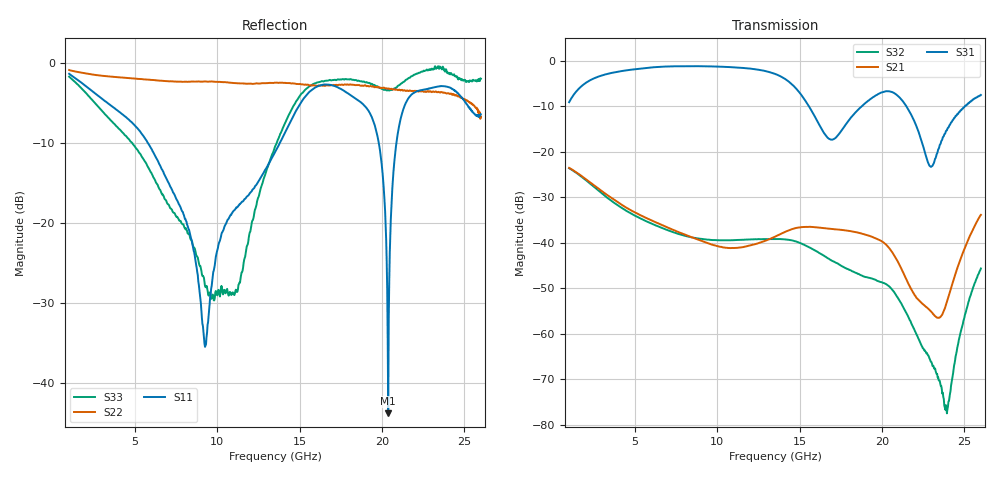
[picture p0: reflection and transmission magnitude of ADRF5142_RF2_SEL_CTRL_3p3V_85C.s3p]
! Device: ADRF5142
! Description: Silicon, SPDT Switch, Reflective
! Frequency: 8.00 GHz - 11.00 GHz
! Ports:
!  RFC = Port 1
!  RF1 = Port 2
!  RF2 = Port 3
! VDD = +3.3V
! VSS = -3.3V
! CTRL = +3.3V
! Temp = 85C
! Data:  Data was collected using an calibrated 4 port network analyzer.
!  The reference plane is the package pins of ADRF5142 switch.
! Notes: Analog Devices supplies this data as a sample of measured data
!  for this product.  Your particular data for this product may vary.
!  Data was taken at 85 degrees C.
!  Analog Devices reserves the right to change this data at anytime.
# HZ S DB R 50
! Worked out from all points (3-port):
!   801 points, 1 GHz to 26 GHz, reference 50 ohm
!   strongest paths, dB at 1 GHz, 7.25 GHz, 13.5 GHz, 19.75 GHz, 26 GHz:
!     S31: -9.1, -1.2, -2.9, -7.3, -7.5
!     S21: -23.5, -37.0, -38.6, -39.2, -33.9
!     S32: -23.6, -37.6, -39.2, -48.4, -45.6
!   lowest |S11| = -43.8 dB at 20.38 GHz (marker M1), VSWR 1.01, Z = 50.2 - j0.611 ohm
!   |S11| at or under -10 dB: 5.768 GHz to 13.8 GHz (8.035 GHz wide, 82.1 % of centre); 19.8 GHz to 20.87 GHz (1.075 GHz wide, 5.29 % of centre)
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1e9  -1.40 158.2  -23.53 -37.4  -9.09 36.3
     -23.53 -37.4  -0.93 171.1  -23.60 -55.0
     -9.09 36.3  -23.60 -55.0  -1.76 124.9
5.8437e9  -10.24 96.3  -34.81 -123.0  -1.49 -86.4
          -34.81 -123.0  -2.14 142.0  -35.52 139.4
          -1.49 -86.4  -35.52 139.4  -13.22 -71.7
9.25e9  -35.52 -51.5  -39.87 -152.3  -1.19 -162.8
        -39.87 -152.3  -2.36 120.3  -39.26 63.2
        -1.19 -162.8  -39.26 63.2  -27.91 -110.1
1.35e10  -11.20 -124.6  -38.64 -171.1  -2.86 90.2
         -38.64 -171.1  -2.51 95.3  -39.16 -38.9
         -2.86 90.2  -39.16 -38.9  -10.51 66.5
1.65e10  -2.73 166.8  -36.79 129.1  -15.99 37.2
         -36.79 129.1  -2.89 75.8  -42.90 -140.1
         -15.99 37.2  -42.90 -140.1  -2.30 -41.9
1.90625e10  -5.69 84.7  -38.28 78.3  -9.04 57.4
            -38.28 78.3  -2.96 62.3  -47.56 142.5
            -9.04 57.4  -47.56 142.5  -2.44 -97.5
2.0375e10  -43.82 -70.7  -40.90 44.5  -6.69 11.1
           -40.90 44.5  -3.24 54.3  -49.41 88.6
           -6.69 11.1  -49.41 88.6  -3.47 -108.5
2.12187e10  -6.31 -176.8  -46.07 28.7  -8.68 -26.4
            -46.07 28.7  -3.41 47.6  -53.71 49.4
            -8.68 -26.4  -53.71 49.4  -2.56 -114.3
2.39062e10  -2.99 63.2  -53.36 150.3  -15.33 20.3
            -53.36 150.3  -3.86 29.0  -76.46 -45.7
            -15.33 20.3  -76.46 -45.7  -0.95 -160.5
2.6e10  -6.46 -42.6  -33.86 144.2  -7.50 -24.9
        -33.86 144.2  -6.77 9.5  -45.65 155.9
        -7.50 -24.9  -45.65 155.9  -2.02 174.3
